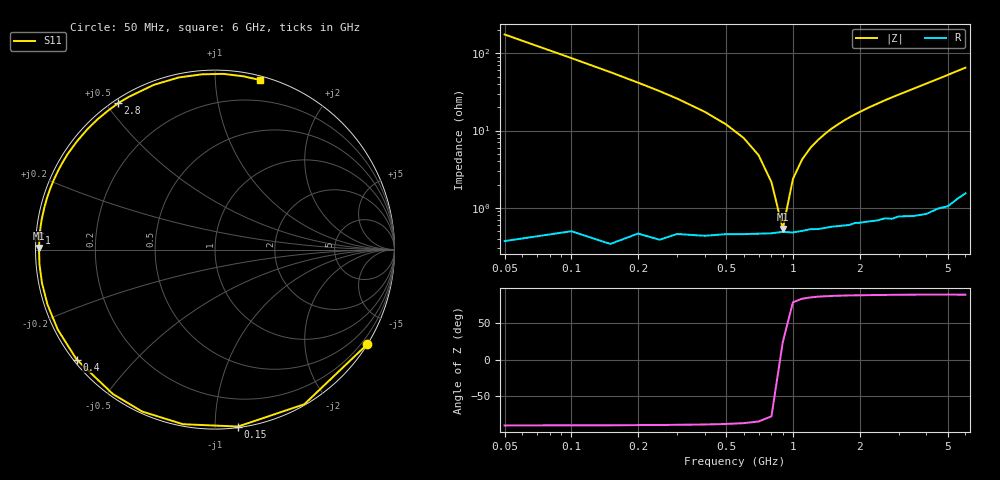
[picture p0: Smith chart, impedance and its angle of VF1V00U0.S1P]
! Infineon Technologies  Discrete & RF Semiconductors
! BBY 58-03
! Si Tuning Diode in SOD323
! VR = 1 V
! S-Parameters:  June  1999
# GHz  S  MA  R  50
!  f  S11
! GHz  MAG  ANG
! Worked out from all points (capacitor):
!   34 points, 50 MHz to 6 GHz, reference 50 ohm
!   read as one part to ground: C = 18.1 pF near 50 MHz
!   lowest |Z| = 534 mohm at 900 MHz (marker M1)
!   series resonance near 890.6 MHz, so ESL is about 1.8 nH
!   S11 on the Smith chart (normalised r, x): 50 MHz: 0.01, -3.50; 150 MHz: 0.01, -1.14; 400 MHz: 0.01, -0.35; 1 GHz: 0.01, +0.05; 2.8 GHz: 0.01, +0.54; 6 GHz: 0.03, +1.30
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0.05  0.9989 -31.9
0.1  0.995 -60.0
0.15  0.9941 -82.6
0.2  0.9891 -100.4
0.25  0.9892 -114.2
0.3  0.9857 -125.2
0.4  0.9846 -141.5
0.5  0.9829 -153.1
0.6  0.9823 -161.9
0.7  0.9819 -169.1
0.8  0.9815 -175.2
0.9  0.9807 179.5
1  0.981 174.7
1.2  0.9794 166.4
1.3  0.9795 162.8
1.6  0.9783 152.9
1.8  0.9782 147.0
2  0.9774 141.7
2.2  0.9772 136.7
2.4  0.9774 132.1
2.8  0.9779 123.5
3  0.9772 119.5
3.5  0.9791 110.4
4  0.9801 101.9
4.5  0.9793 94.3
5  0.9802 87.3
5.5  0.9785 80.8
6  0.9774 75.1
